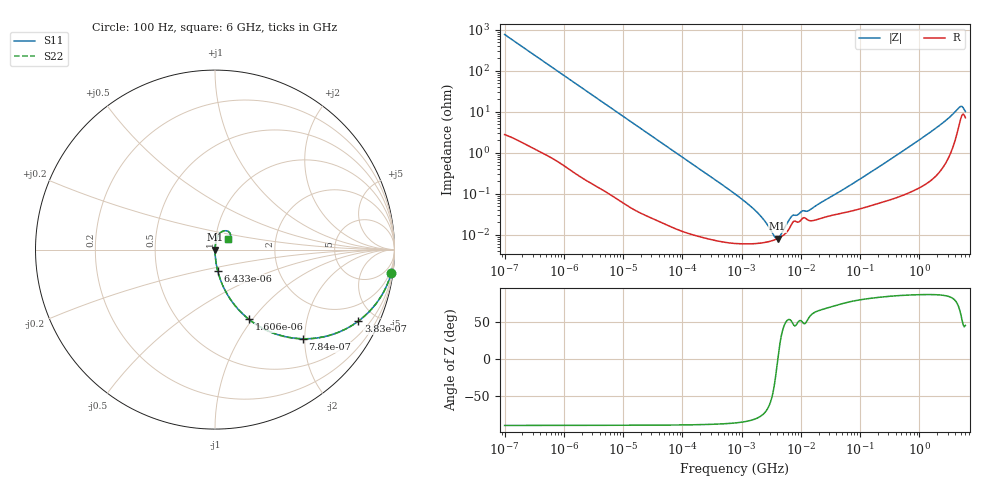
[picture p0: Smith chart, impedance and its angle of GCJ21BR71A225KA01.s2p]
!Murata Part Number: GCJ21BR71A225KA01
!These Parameters are Measured in Series Mode Connection
!Data Generated on Mar 13, 2026
!  o--ll--o
!Port1  Port2
!  o------o
!Operation Temp=25[degC], DC Bias Voltage=0[V]
!Freq. Start=100[Hz] Stop=6[GHz] 401[Steps]
# Hz S RI R 50
!Freq.(Hz) S11(Real) S11(Imag) S21(Real) S21(Imag) S12(Real) S12(Imag) S22(Real) S22(Imag)
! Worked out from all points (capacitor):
!   401 points, 100 Hz to 6 GHz, reference 50 ohm
!   read as one part in series: C = 2.08 uF near 109 Hz
!   lowest |Z| = 8.08 mohm at 4.06 MHz (marker M1)
!   series resonance near 4.096 MHz, so ESL is about 720 pH
!   S11 on the Smith chart (normalised r, x): 100 Hz: 1, -15; 383 Hz: 1.02, -4.00; 784 Hz: 1.01, -1.96; 1.606 kHz: 1.01, -0.96; 6.433 kHz: 1.00, -0.24; 6 GHz: 1.14, +0.14
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100  0.9827 -0.1287  0.0173 0.1287  0.0173 0.1287  0.9827 -0.1287
214  0.9263 -0.259  0.0737 0.259  0.0737 0.259  0.9263 -0.259
383  0.7986 -0.3983  0.2014 0.3983  0.2014 0.3983  0.7986 -0.3983
784  0.4898 -0.4968  0.5102 0.4968  0.5102 0.4968  0.4898 -0.4968
1606  0.1888 -0.3882  0.8112 0.3882  0.8112 0.3882  0.1888 -0.3882
2008  0.1301 -0.3333  0.8699 0.3333  0.8699 0.3333  0.1301 -0.3333
6433  0.0152 -0.1186  0.9848 0.1186  0.9848 0.1186  0.0152 -0.1186
40335  0.000586 -0.0194  0.9994 0.0194  0.9994 0.0194  0.000586 -0.0194
774597  6.23e-05 -0.000989  0.9999 0.000989  0.9999 0.000989  6.23e-05 -0.000989
1734173  6.12e-05 -0.000377  0.9999 0.000377  0.9999 0.000377  6.12e-05 -0.000377
2372521  6.45e-05 -0.000223  0.9999 0.000223  0.9999 0.000223  6.45e-05 -0.000223
3394479  7.29e-05 -7.39e-05  0.9999 7.39e-05  0.9999 7.39e-05  7.29e-05 -7.39e-05
4060267  8.07e-05 -3.4e-06  0.9999 3.4e-06  0.9999 3.4e-06  8.07e-05 -3.4e-06
4856642  9.32e-05 6.83e-05  0.9999 -6.83e-05  0.9999 -6.83e-05  9.32e-05 6.83e-05
6353432  0.00014 0.000184  0.9999 -0.000184  0.9999 -0.000184  0.00014 0.000184
7266822  0.000198 0.000219  0.9998 -0.000219  0.9998 -0.000219  0.000198 0.000219
1.555665e7  0.00022 0.000384  0.9998 -0.000384  0.9998 -0.000384  0.00022 0.000384
3.124326e8  0.000744 0.00659  0.9993 -0.00659  0.9993 -0.00659  0.000744 0.00659
1.95892e9  0.00446 0.0406  0.9955 -0.0406  0.9955 -0.0406  0.00446 0.0406
4.586474e9  0.0507 0.1048  0.9493 -0.1048  0.9493 -0.1048  0.0507 0.1048
5.245841e9  0.0847 0.0904  0.9153 -0.0904  0.9153 -0.0904  0.0847 0.0904
6e9  0.0707 0.0614  0.9293 -0.0614  0.9293 -0.0614  0.0707 0.0614
